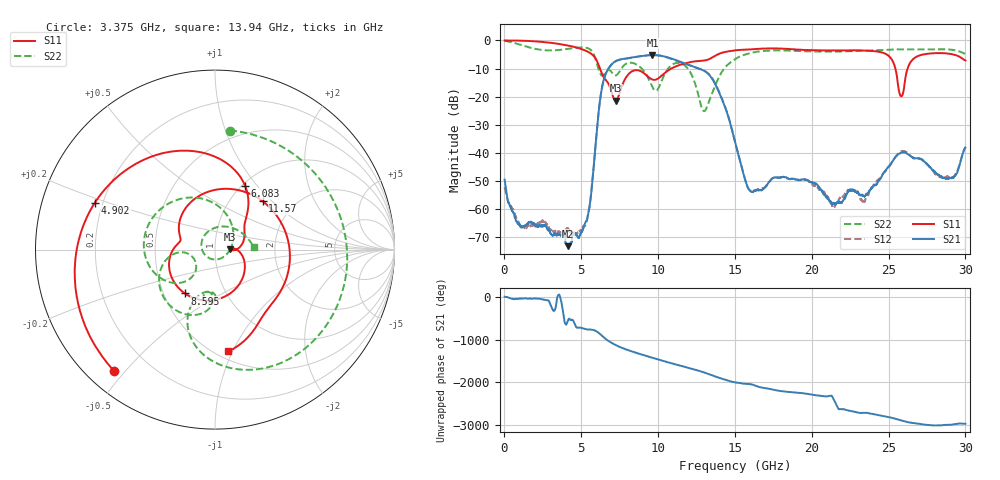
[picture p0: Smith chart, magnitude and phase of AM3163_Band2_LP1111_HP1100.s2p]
!Agilent Technologies,E8364B,MY43040894,A.07.50.67
!Agilent E8364B: A.07.50.67
!Date: Thursday, August 20, 2020 12:08:33
!Correction: S11(Full 2 Port(1,2))
!S21(Full 2 Port(1,2))
!S12(Full 2 Port(1,2))
!S22(Full 2 Port(1,2))
!S2P File: Measurements: S11, S21, S12, S22:
# Hz S  dB  R 50
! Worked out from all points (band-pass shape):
!   3201 points, 10 MHz to 30 GHz, reference 50 ohm
!   highest |S21| = -5.21 dB at 9.635 GHz (marker M1); lowest = -73.1 dB at 4.143 GHz (marker M2)
!   |S21| within 3 dB of the highest: 7.033 GHz to 11.75 GHz (4.721 GHz wide, 50.3 % of centre)
!   lowest |S11| = -21.4 dB at 7.245 GHz (marker M3), VSWR 1.19, Z = 59.3 + j0.248 ohm
!   |S11| at or under -10 dB: 6.215 GHz to 10.86 GHz (4.645 GHz wide, 54.4 % of centre); 25.44 GHz to 26.24 GHz (795.5 MHz wide, 3.08 % of centre)
!   |S22| runs from -25.1 to -0.2 dB; largest |S21 - S12| = 0.011
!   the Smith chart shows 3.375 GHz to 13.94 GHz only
!   S11 on the Smith chart (normalised r, x): 3.375 GHz: 0.08, -0.47; 4.902 GHz: 0.17, +0.18; 6.083 GHz: 1.03, +0.87; 8.595 GHz: 0.64, -0.34; 11.57 GHz: 1.40, +0.88; 13.94 GHz: 0.57, -0.96
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1e7  -0.03 -2.8  -49.47 6.0  -52.11 17.8  -0.18 -6.9
1.790656e9  -0.28 -67.7  -64.75 -40.2  -65.56 5.0  -2.74 -158.8
3.374503e9  -1.12 -129.9  -68.71 -153.8  -67.94 66.4  -3.50 82.9
4.142997e9  -1.84 -163.1  -73.10 172.3  -67.02 179.6  -3.01 30.1
4.902119e9  -2.87 158.6  -69.35 0.2  -67.62 -2.8  -2.52 -21.9
5.014581e9  -3.08 152.1  -68.22 -7.6  -67.24 -8.8  -2.50 -30.0
6.082975e9  -8.11 64.8  -27.91 -108.1  -27.98 -108.4  -9.55 -113.0
7.245088e9  -21.40 1.4  -7.36 -46.8  -7.40 -46.8  -12.43 -98.3
8.594638e9  -10.56 -124.4  -5.82 129.7  -5.84 130.0  -8.56 -145.3
9.634916e9  -13.92 167.7  -5.21 16.0  -5.21 16.0  -16.62 -170.2
1.000979e10  -13.50 158.2  -5.32 -23.9  -5.33 -24.2  -17.09 -138.5
1.156552e10  -8.45 45.3  -7.82 179.7  -7.96 -179.0  -8.33 147.0
1.29713e10  -7.18 -43.8  -10.74 36.0  -10.71 37.5  -25.10 -85.8
1.393661e10  -4.85 -82.5  -18.10 -87.8  -17.81 -87.4  -13.33 3.4
1.5005e10  -3.56 -131.5  -36.19 161.2  -36.17 160.4  -6.70 -112.2
1.600779e10  -3.19 -173.8  -53.60 118.6  -53.49 117.5  -4.50 -172.5
1.787279e10  -2.89 98.3  -48.87 -36.3  -48.65 -35.6  -3.57 92.2
2.000958e10  -3.50 -9.8  -50.28 -124.9  -51.05 -121.1  -3.94 -9.3
2.230569e10  -3.55 -99.8  -54.26 -131.7  -53.56 -137.3  -3.86 -93.5
2.500479e10  -5.49 157.5  -44.73 68.0  -44.94 70.8  -3.35 -167.5
2.582014e10  -19.85 170.3  -39.92 -8.4  -39.40 -7.4  -3.20 170.4
3e10  -7.14 51.1  -38.06 -89.6  -37.95 -86.4  -4.83 55.5
